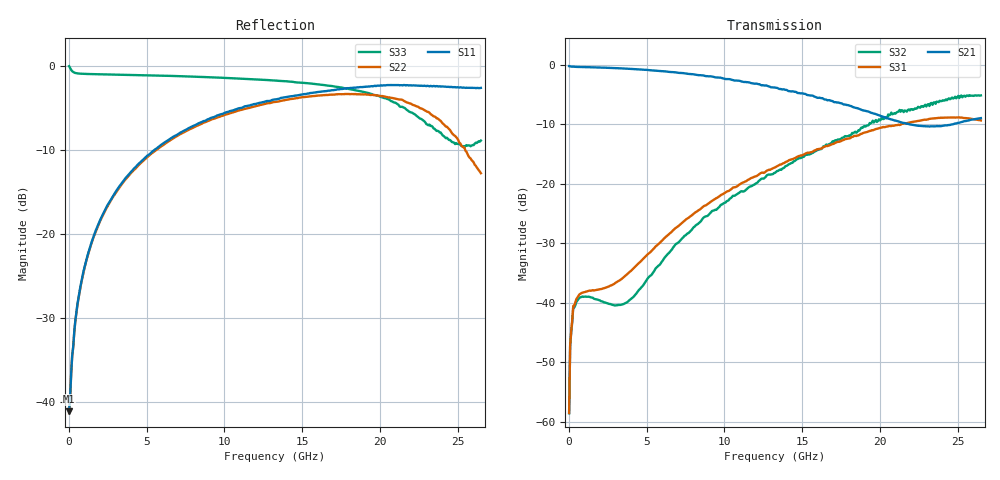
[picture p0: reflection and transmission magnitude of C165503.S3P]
!  3-Port S-parameters saved by WinCal
! VAR MeasName=S-Parameters (CALIBRATED_DATA) read from VNA (N5242A)
! VAR MeasDate=2016-5-24 8:48:57
! VAR NAME=C165503
! VAR FILENAME=C165503.S3P
! VAR DATE=2016-5-24 8:48:57
! VAR PHYS_PORTS=1,2,3
! VAR ObjTypeName=DATASET
! VAR IndexType=Frequency
# Hz S DB R 50
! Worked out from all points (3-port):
!   401 points, 10 MHz to 26.5 GHz, reference 50 ohm
!   strongest paths, dB at 10 MHz, 6.633 GHz, 13.26 GHz, 19.88 GHz, 26.5 GHz:
!     S21: -0.2, -1.2, -3.8, -8.4, -8.9
!     S31: -58.5, -28.0, -17.2, -10.7, -9.3
!     S32: -58.6, -31.0, -18.1, -9.4, -5.1
!   lowest |S11| = -41.1 dB at 10 MHz (marker M1), VSWR 1.02, Z = 50.8 - j0.282 ohm
!   |S11| at or under -10 dB: start of sweep to 5.508 GHz
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1e7  -41.12 -18.4  -0.21 -0.2  -60.28 56.6
     -0.21 -0.3  -41.34 -19.1  -60.48 65.0
     -58.49 44.4  -58.55 45.3  -0.05 -6.1
2.08675e8  -34.47 -97.2  -0.29 -1.7  -43.01 44.3
           -0.29 -1.7  -34.48 -98.5  -43.29 40.8
           -42.96 45.4  -43.27 41.6  -0.65 -94.6
4.0735e8  -30.38 -102.2  -0.32 -2.9  -40.00 36.2
          -0.32 -2.9  -30.39 -103.2  -40.42 31.1
          -39.93 36.5  -40.41 31.3  -0.86 -130.1
1.0696e9  -23.43 -102.9  -0.37 -6.8  -38.22 29.7
          -0.37 -6.8  -23.52 -104.5  -39.03 18.9
          -38.13 29.9  -38.94 19.0  -0.97 -163.1
3.4537e9  -13.83 -111.5  -0.60 -21.2  -35.92 65.0
          -0.60 -21.1  -13.96 -115.2  -40.27 49.8
          -35.82 65.1  -40.24 50.1  -1.07 174.1
5.17555e9  -10.53 -120.3  -0.89 -31.7  -31.73 84.6
           -0.88 -31.5  -10.66 -125.5  -35.58 82.8
           -31.60 84.8  -35.55 82.8  -1.14 165.9
1.3255e10  -4.00 -161.4  -3.94 -75.6  -17.34 76.2
           -3.80 -75.9  -4.31 -176.4  -18.05 62.5
           -17.23 75.8  -18.14 62.3  -1.76 132.9
1.742718e10  -2.79 179.5  -6.45 -93.0  -12.97 55.4
             -6.40 -92.9  -3.39 155.7  -12.48 33.0
             -12.86 55.5  -12.50 33.0  -2.57 114.0
2.14669e10  -2.34 160.2  -10.17 -100.1  -10.25 29.6
            -9.74 -98.4  -4.08 123.8  -8.05 -11.1
            -9.88 28.7  -7.65 -12.4  -4.90 93.9
2.65e10  -2.63 141.9  -8.97 -94.8  -9.37 -10.0
         -8.94 -95.0  -12.79 112.4  -5.12 -70.0
         -9.32 -10.1  -5.12 -70.1  -8.90 116.9
